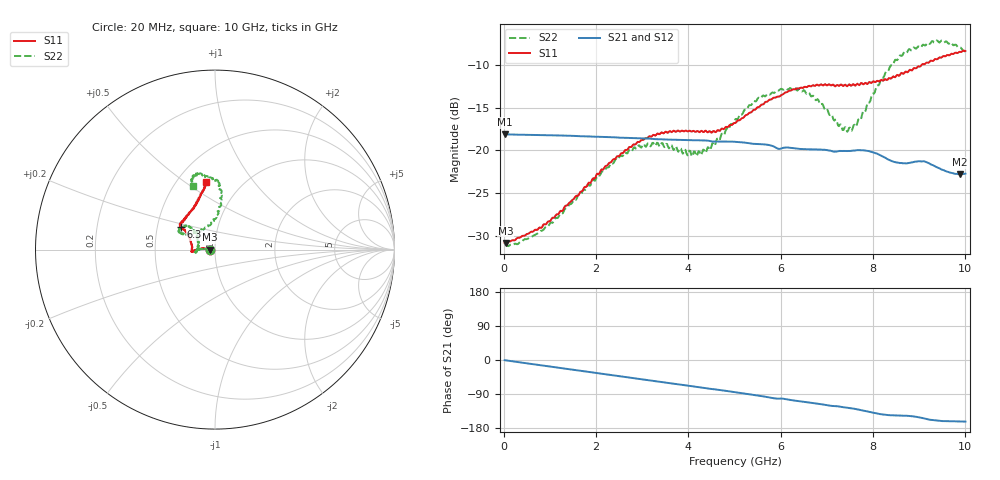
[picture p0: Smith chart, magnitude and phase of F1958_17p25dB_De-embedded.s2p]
! Integrated Device Technology
! Corporate Headquarters
! 6024 Silver Creek Valley Road
! San Jose, CA 95138  USA
! Phone:  1-408-284-8200
! Toll Free:  1-800-223-1366
! Webpage:  http://www.idt.com/
! Timing and RF Division
! 515 Groton Road, Suite 102
! Westford, MA 01886-6024
! Device:  F1958
! Description: 7-bit 0.25 dB Digital Step Attenuator
! Frequency:  0.001 -  6.000 GHz
! Package:  4x4 mm Thin QFN Plastic Package: 24 pin
! Ports:  2 RF, 12 DC
!  Pin  1  = D0
!  Pin  2  = VDD
!  Pin  3  = VMODE
!  Pin  4  = GND
!  Pin  5  = RF1  =  Port 1
!  Pin  6  = GND
!  Pin  7  = GND
!  Pin  8  = GND
!  Pin  9  = GND
!  Pin 10  = GND
!  Pin 11  = GND
!  Pin 12  = GND
!  Pin 13  = GND
!  Pin 14  = RF2  =  Port 2
!  Pin 15  = GND
!  Pin 16  = LE
!  Pin 17  = CLK
!  Pin 18  = DATA
!  Pin 19  = D6
!  Pin 20  = D5
!  Pin 21  = D4
!  Pin 22  = D3
!  Pin 23  = D2
!  Pin 24  = D1
! State:  69
! Atten State:  17.25 dB
! Voltage:  +3.30 Volts
! Current:  0.258 mA
! Data:  The device was measured on a F1958 evaluation board which has
!  individual transmission lines to the RF pins.  Data was collected
!  using a calibrated network analyzer.  The evaluation board was
!  de-embedded using Automatic Fixture Removal (AFR).
!  The reference plane is the edge of the package pin.
! Misc:
!  Action Tracker AT0419
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# GHz S dB R 50
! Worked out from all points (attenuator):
!   500 points, 20 MHz to 10 GHz, reference 50 ohm
!   highest |S21| = -18.12 dB at 20 MHz (marker M1); lowest = -22.8 dB at 9.88 GHz (marker M2)
!   lowest |S11| = -30.8 dB at 40 MHz (marker M3), VSWR 1.06, Z = 47.2 - j0.0652 ohm
!   |S11| at or under -10 dB: start of sweep to 9.057 GHz
!   |S22| runs from -31.1 to -7.2 dB; largest |S21 - S12| = 0.00045
!   S11 on the Smith chart (normalised r, x): 20 MHz: 0.94, -0.00; 6.3 GHz: 0.66, +0.17; 10 GHz: 0.69, +0.60
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0.02  -30.74 -178.6  -18.12 -0.5  -18.11 -0.4  -30.97 -178.8
0.04  -30.76 -178.6  -18.12 -0.8  -18.12 -0.8  -30.94 -178.2
0.32  -30.17 176.9  -18.16 -5.7  -18.16 -5.7  -30.84 176.9
0.84  -28.84 174.4  -18.21 -14.5  -18.20 -14.5  -29.31 176.2
1.7  -24.74 175.1  -18.35 -29.1  -18.34 -29.1  -24.83 175.0
2.6  -20.20 179.4  -18.52 -44.3  -18.50 -44.3  -20.44 -179.4
2.92  -19.01 -177.5  -18.58 -49.8  -18.56 -49.8  -19.41 -175.8
3.36  -18.10 -174.7  -18.69 -57.2  -18.69 -57.4  -19.39 -171.4
4.24  -17.88 -179.5  -18.82 -71.9  -18.84 -71.9  -20.13 166.8
4.5  -17.93 174.6  -18.94 -76.6  -18.95 -76.6  -19.50 151.5
5.02  -16.79 160.2  -18.99 -85.2  -19.00 -85.2  -16.34 138.5
5.56  -14.78 149.6  -19.26 -94.8  -19.28 -94.8  -13.95 139.6
6.3  -12.89 146.6  -19.75 -107.1  -19.75 -107.0  -12.71 151.6
6.68  -12.45 144.6  -19.87 -113.1  -19.89 -113.0  -13.68 153.3
7.3  -12.32 138.4  -20.06 -123.4  -20.06 -123.4  -16.97 132.8
7.5  -12.36 135.7  -20.06 -126.9  -20.06 -126.8  -17.34 114.8
7.7  -12.40 131.6  -19.96 -131.2  -19.96 -131.2  -16.34 98.4
8.34  -11.59 116.6  -21.08 -145.5  -21.08 -145.7  -10.63 82.9
8.68  -10.95 110.1  -21.50 -147.0  -21.50 -146.9  -8.51 87.2
9.26  -9.54 102.4  -21.65 -158.1  -21.64 -158.1  -7.38 99.8
9.88  -8.51 98.1  -22.75 -162.1  -22.80 -162.0  -7.98 108.6
10  -8.42 97.8  -22.69 -162.6  -22.73 -162.5  -8.50 109.2
